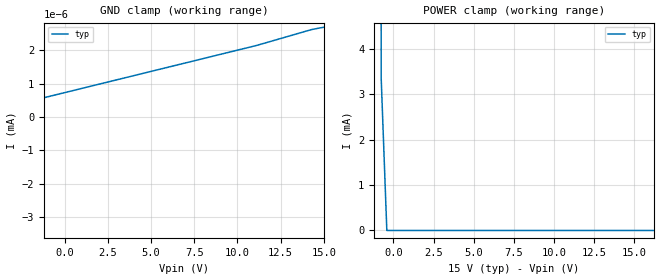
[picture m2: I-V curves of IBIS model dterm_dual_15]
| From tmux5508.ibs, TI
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| dterm_dual_15
[Model]   dterm_dual_15
Model_type   Terminator
|   typ   min   max
C_comp   1.008417e-11   NA   NA
[Voltage Range]   15   NA   NA
[Temperature Range]   27   NA   NA
[Power Clamp Reference]   15   NA   NA
[GND Clamp Reference]   0   NA   NA
[GND Clamp]
|   Voltage   I(typ)   I(min)   I(max)
-20V      -2.839A    NA         NA
-15.4V    -221.5nA   NA         NA
-15.05V   -1.213nA   NA         NA
-14.34V   -1.14nA    NA         NA
-11.16V   -686pA     NA         NA
11.11V    2.144nA    NA         NA
14.29V    2.618nA    NA         NA
15V       2.688nA    NA         NA
[POWER Clamp]
|   Voltage   I(typ)   I(min)   I(max)
-5V       8.449A     NA         NA
-1.111V   238.4mA    NA         NA
-757.6mV  3.381mA    NA         NA
-404mV    187.2nA    NA         NA
30V       -3.229nA   NA         NA
